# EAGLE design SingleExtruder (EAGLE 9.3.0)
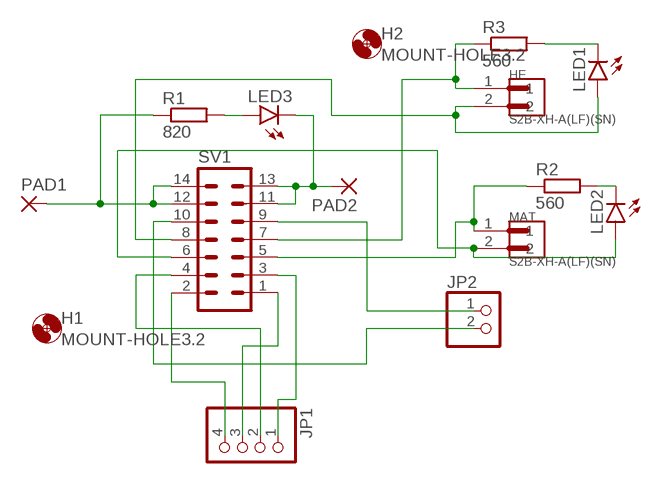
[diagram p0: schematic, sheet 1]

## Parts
H1  MOUNT-HOLE3.2  [3,2]
H2  MOUNT-HOLE3.2  [3,2]
HE  S2B-XH-A(LF)(SN)  [JST_S2B-XH-A(LF)(SN)]
JP1  PINHD-1X4/90  [1X04/90]
JP2  PINHD-1X2/90  [1X02/90]
LED1  LEDCHIPLED_0805  [CHIPLED_0805]
LED2  LEDCHIPLED_0805  [CHIPLED_0805]
LED3  LEDCHIPLED_0805  [CHIPLED_0805]
MAT  S2B-XH-A(LF)(SN)  [JST_S2B-XH-A(LF)(SN)]
PAD1  SMD5  [SMD2,54-5,08]
PAD2  SMD5  [SMD2,54-5,08]
R1  820  R-EU_R0805  [R0805]
R2  560  R-EU_R0805  [R0805]
R3  560  R-EU_R0805  [R0805]
SV1  ML14  [ML14]

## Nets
E_A+: JP1.4 SV1.2
E_A-: JP1.3 SV1.1
E_B+: JP1.2 SV1.4
E_B-: JP1.1 SV1.3
F0: MAT.1 R2.1 SV1.5
F0_VCC: LED2.A MAT.2 SV1.6
F1: HE.1 R3.1 SV1.7
F1_VCC: HE.2 LED1.A SV1.8
H0: LED3.C PAD2.1(P) SV1.11 SV1.13
N$1: LED3.A R1.2
N$12: LED1.C R3.2
N$14: LED2.C R2.2
T_H0_A: JP2.1 SV1.9
T_H0_B: JP2.2 SV1.10
VCC: PAD1.1(P) R1.1 SV1.12 SV1.14

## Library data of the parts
H1 H2 = holes:MOUNT-HOLE: MOUNTING HOLE with drill center marker
HE MAT = S2B-XH-A_LF__SN_:S2B-XH-A(LF)(SN): XH Series 2.5mm 2 Position Through Hole Shrouded Header Connector; AVAILABILITY: Unavailable; DESCRIPTION: XH Series 2.5mm 2 Position Through Hole Shrouded Header Connector; MF: JST Sales; MP: S2B-XH-A_LF__SN_; PACKAGE: FakePackage u; PRICE: None
JP1 = pinhead:PINHD-1X4: PIN HEADER
JP2 = pinhead:PINHD-1X2: PIN HEADER
LED1-LED3 = led:LED: LED
PAD1 PAD2 = wirepad:SMD5: SMD PAD
R1-R3 = resistor:R-EU_: RESISTOR, European symbol
SV1 = con-harting-ml:ML14: HARTING; OC_FARNELL: unknown; OC_NEWARK: unknown

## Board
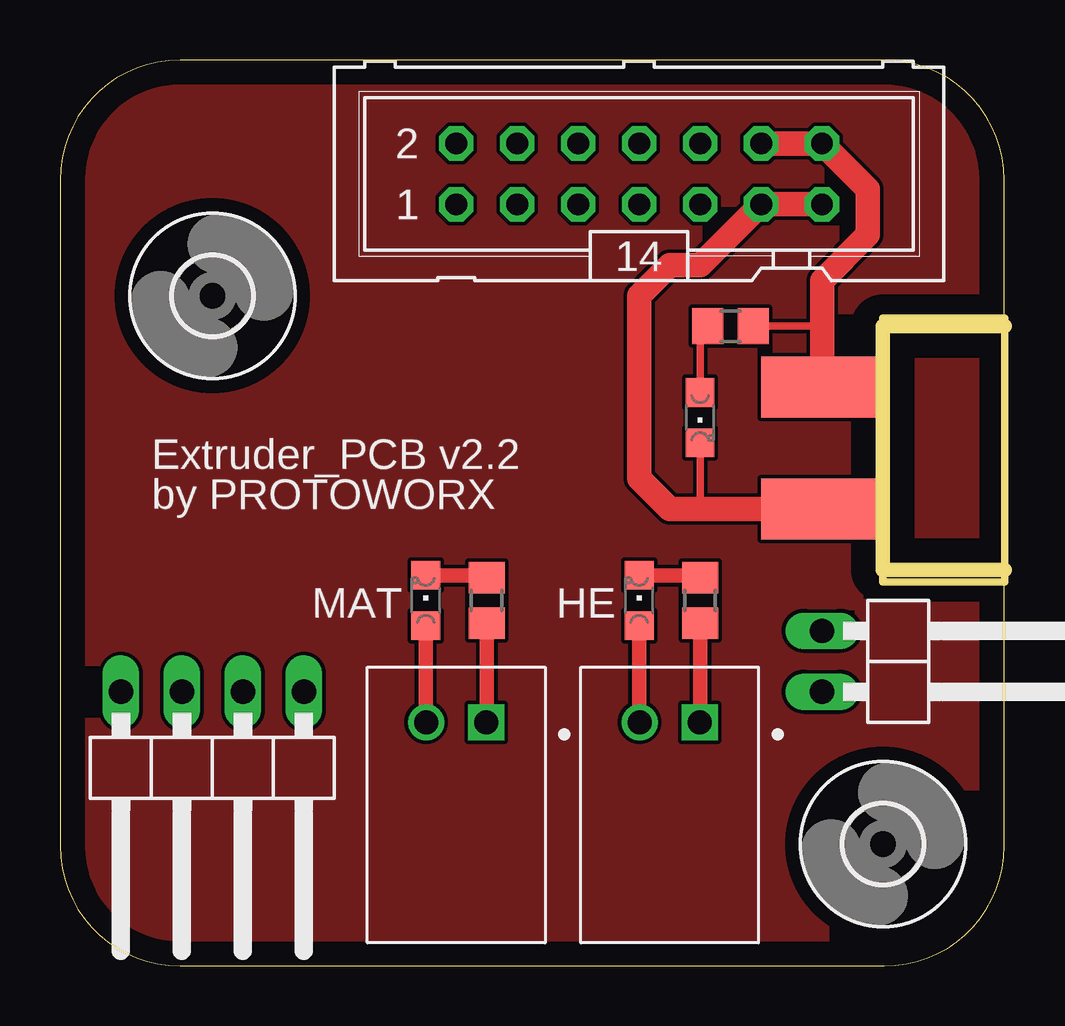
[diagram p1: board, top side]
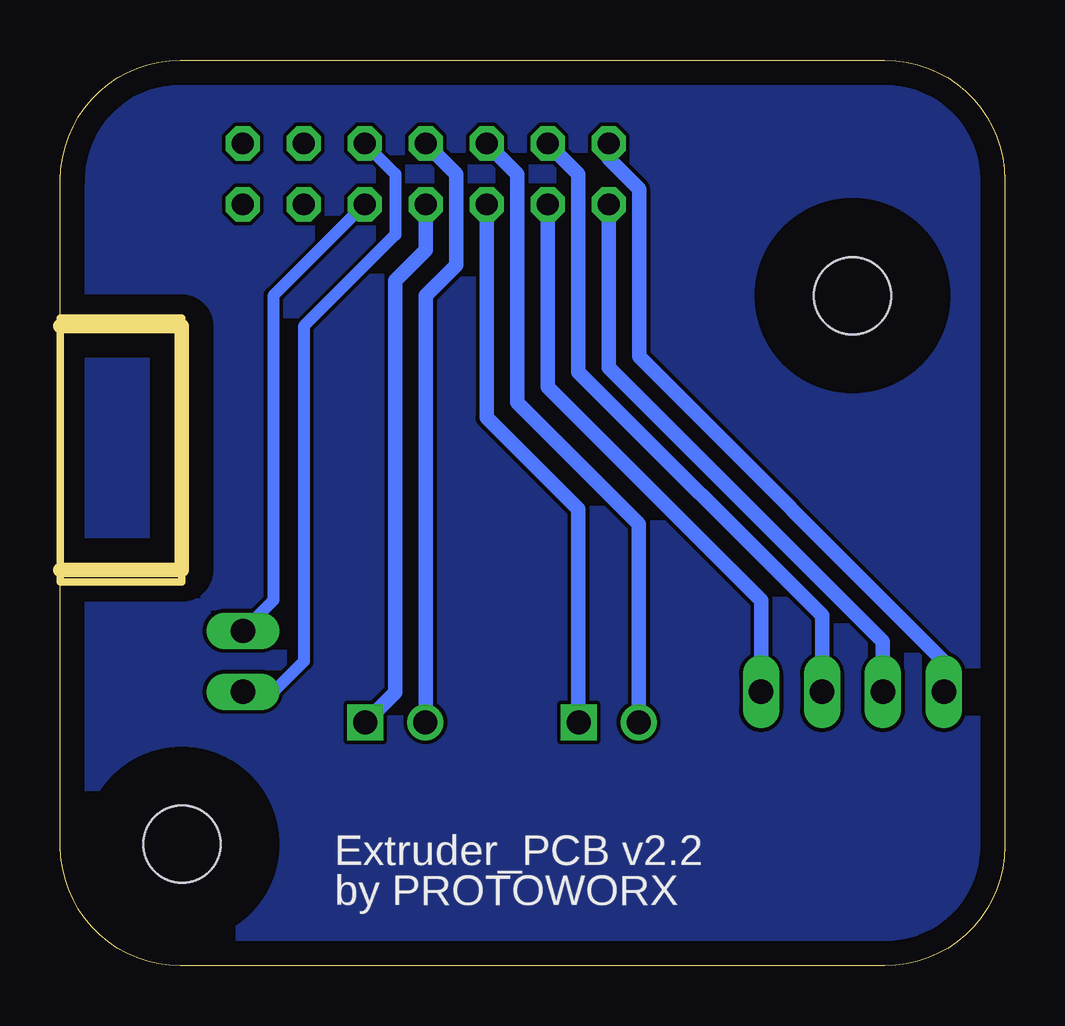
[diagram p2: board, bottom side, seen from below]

Size 39.37 x 37.77 mm. Coordinates in mm from the lower left corner, seen from the top.
Outline: 39.37,26.67 34.29,26.67 34.29,16.51 39.37,16.51
Outline: 0,32.77 0,5 arc90 5,0 34.35,0 arc90 39.35,5 39.35,32.77 arc90 34.35,37.77 5,37.77 arc90 0,32.77
Copper layers (1*16): Top 0.035mm / dielectric 1.5mm / Bottom 0.035mm
Design rules "default": minimum track width 6mil, minimum drill 0.35mm, track to track 6mil, track to pad 6mil, pad to pad 6mil, via to via 6mil, smd to smd 6mil, copper to edge 40mil, drill to drill 6mil, minimum pad ring 10mil, minimum via ring 8mil, stop-mask expansion 4mil, vias tented up to drill 0mil, thermal gap 10mil
Milling: 4 lines

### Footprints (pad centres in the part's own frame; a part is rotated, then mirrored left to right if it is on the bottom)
3,2 = hole 3.2: 0,0
JST_S2B-XH-A(LF)(SN) = drill 1 square: 1 -1.25,0 | drill 1: 2 1.25,0
1X04/90 = drill 1.016 long: 1 -3.81,-3.81; 2 -1.27,-3.81; 3 1.27,-3.81; 4 3.81,-3.81
1X02/90 = drill 1.016 long: 1 -1.27,-3.81; 2 1.27,-3.81
CHIPLED_0805 = smd 1.2 x 1.2: A 0,-1.05; C 0,1.05
SMD2,54-5,08 = smd 2.54 x 5.08: 1 0,0
R0805 = smd 1.3 x 1.5: 1 -0.95,0; 2 0.95,0
ML14 = drill 0.914 octagon: 1 -7.62,-1.27; 2 -7.62,1.27; 3 -5.08,-1.27; 4 -5.08,1.27; 5 -2.54,-1.27; 6 -2.54,1.27; 7 0,-1.27; 8 0,1.27; 9 2.54,-1.27; 10 2.54,1.27; 11 5.08,-1.27; 12 5.08,1.27; 13 7.62,-1.27; 14 7.62,1.27

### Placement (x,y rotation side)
H1  34.29,5.08 0 top
H2  6.35,27.94 0 top
HE  25.4,10.16 180 top
JP1  6.35,7.62 180 top
JP2  35.56,12.7 270 top
LED1  24.13,15.24 0 top
LED2  15.24,15.24 0 top
LED3  26.67,22.86 180 top
MAT  16.51,10.16 180 top
PAD1  31.75,24.13 90 top
PAD2  31.75,19.05 90 top
R1  27.94,26.67 180 top
R2  17.78,15.24 90 top
R3  26.67,15.24 90 top
SV1  24.13,33.02 0 top

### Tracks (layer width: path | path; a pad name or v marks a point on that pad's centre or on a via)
E_A+
  Bottom 0.61: SV1.2 16.51,33.66 15.24,32.38 15.24,25.4 2.54,12.7 JP1.4
E_A-
  Bottom 0.61: JP1.3 5.08,13.53 16.51,24.96 SV1.1
E_B+
  Bottom 0.61: SV1.4 17.78,33.02 17.78,24.77 7.62,14.61 JP1.2
E_B-
  Bottom 0.61: SV1.3 19.05,24.13 10.16,15.24 JP1.1
F0
  Top 0.61: R2.1 17.78,10.18 MAT.1
  Bottom 0.61: SV1.5 21.59,22.86 17.78,19.05 17.78,10.18
  Bottom 0.813: 17.78,10.18 MAT.1
F0_VCC
  Top 0.61: MAT.2 15.24,10.18 LED2.A
  Bottom 0.61: SV1.6 20.32,33.02 20.32,23.5 15.26,18.43 MAT.2
F1
  Top 0.61: R3.1 26.67,10.18 HE.1
  Bottom 0.61: SV1.7 24.13,29.84 25.4,28.57 25.4,11.41 HE.1
F1_VCC
  Top 0.61: HE.2 24.13,10.18 LED1.A
  Bottom 0.61: SV1.8 22.86,33.02 22.86,29.21 24.13,27.94 24.13,10.16 HE.2
GND
  pour Bottom: 0,33.1 0,5 arc90 5,0 34.37,0 arc90 39.37,5 39.37,33.1 arc90 34.37,38.1 5,38.1 arc90
  pour Top: 0,33.1 0,5 arc90 5,0 34.37,0 arc90 39.37,5 39.37,33.1 arc90 34.37,38.1 5,38.1 arc90
H0
  Top 0.305: LED3.C 26.67,19.05
  Top 1.016: SV1.13 SV1.11 26.67,29.21 25.4,29.21 24.13,27.94 24.13,20.32 25.4,19.05 26.67,19.05 30.48,19.05
  Top 1.27: 30.48,19.05 PAD2.1
N$1
  Top 0.305: LED3.A 26.67,26.35 R1.2
N$12
  Top 0.61: LED1.C 26.57,16.29 R3.2
N$14
  Top 0.61: LED2.C 17.68,16.29 R2.2
T_H0_A
  Bottom 0.508: SV1.9 30.48,27.94 30.48,15.24 JP2.1
T_H0_B
  Bottom 0.508: SV1.10 25.4,33.02 25.4,30.48 29.21,26.67 29.21,12.7 30.48,11.43 JP2.2
VCC
  Top 0.305: R1.1 31.75,26.67
  Top 1.016: PAD1.1 31.75,26.67 31.75,28.57 33.66,30.48 33.66,32.38 SV1.14 SV1.12

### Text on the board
tNames: Extruder_PCB v2.2 / by PROTOWORX
bNames: Extruder_PCB v2.2 / by PROTOWORX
